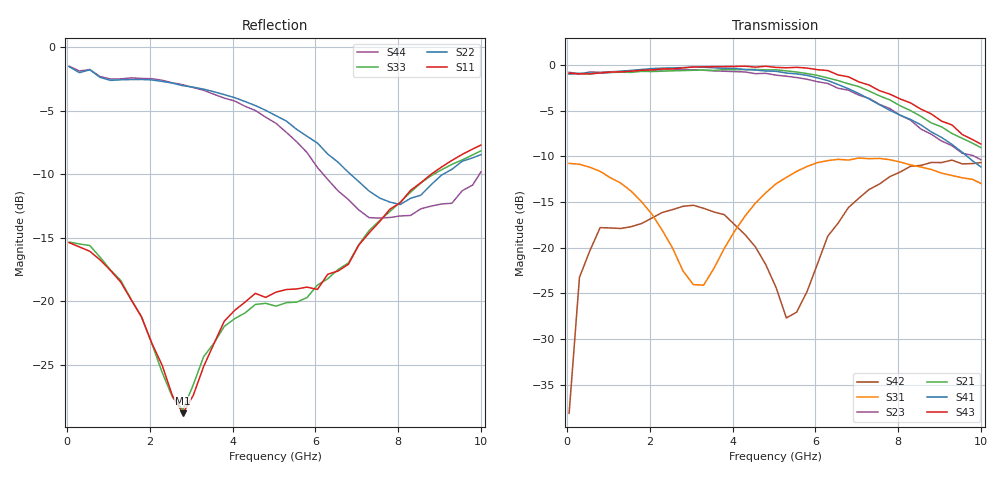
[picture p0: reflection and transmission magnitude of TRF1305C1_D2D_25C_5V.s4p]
! Created Tue Jun 24 22:55:10 2025
# hz S ma R 50
! 4 Port Network Data from SP1.SP block
! PORT[1] = INP
! PORT[2] = OUTM
! PORT[3] = INM
! PORT[4] = OUTP
! freq  magS11  angS11  magS12  angS12  magS13  angS13  magS14  angS14
!  magS21  angS21  magS22  angS22  magS23  angS23  magS24  angS24
!  magS31  angS31  magS32  angS32  magS33  angS33  magS34  angS34
!  magS41  angS41  magS42  angS42  magS43  angS43  magS44  angS44
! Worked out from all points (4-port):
!   41 points, 50 MHz to 10 GHz, reference 50 ohm
!   strongest paths, dB at 50 MHz, 2.55 GHz, 5.05 GHz, 7.55 GHz, 10 GHz:
!     S43: -0.9, -0.4, -0.3, -2.8, -8.7
!     S41: -1.0, -0.3, -0.7, -4.3, -11.2
!     S21: -0.9, -0.6, -0.5, -3.4, -9.0
!     S23: -0.8, -0.5, -1.1, -4.3, -10.4
!     S31: -10.8, -20.0, -13.0, -10.2, -13.0
!     S42: -38.1, -15.8, -24.4, -13.0, -10.7
!   lowest |S11| = -28.8 dB at 2.8 GHz (marker M1), VSWR 1.08, Z = 53.6 - j1.19 ohm
!   |S11| at or under -10 dB: start of sweep to 8.804 GHz
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5e7  0.1699 -1.5  0.004897 20.4  0.2954 -2.0  0.001261 -133.2
     0.8981 178.1  0.8368 178.4  0.9136 -2.0  0.01182 113.1
     0.2894 -2.0  0.00399 98.6  0.1708 -0.8  0.002537 18.8
     0.8926 -1.9  0.0124 122.8  0.9028 177.5  0.8406 178.9
5.5e8  0.1571 -19.1  0.02789 65.3  0.2843 -21.0  0.01899 71.4
       0.8943 157.8  0.8135 164.5  0.9165 -21.4  0.09531 68.9
       0.2758 -20.8  0.02184 69.4  0.1655 -17.2  0.02609 63.2
       0.9017 -20.8  0.09612 68.0  0.8947 158.0  0.8156 166.4
2.8e9  0.03619 -17.8  0.05857 -19.5  0.07844 -128.2  0.03886 -43.8
       0.9327 63.8  0.7042 121.2  0.9438 -112.6  0.1678 -1.2
       0.07477 -129.9  0.04105 -47.5  0.0374 -7.6  0.06172 -15.9
       0.9682 -109.4  0.1686 -4.4  0.9645 65.5  0.7104 128.2
4.3e9  0.09906 17.4  0.07177 -59.6  0.1466 91.2  0.04265 -103.5
       0.9454 -0.4  0.6104 91.4  0.917 -175.3  0.1241 -46.2
       0.1489 88.7  0.04447 -105.4  0.08983 22.8  0.07748 -55.3
       0.9445 -174.0  0.118 -52.5  0.9861 2.4  0.5844 97.9
6.05e9  0.1112 3.5  0.09128 -108.9  0.2992 33.5  0.03464 175.1
        0.8776 -80.8  0.4189 58.9  0.8106 103.1  0.06619 111.8
        0.2923 31.5  0.03239 177.4  0.1157 16.1  0.09526 -106.3
        0.8507 104.2  0.08138 115.8  0.943 -78.0  0.3357 67.4
7.8e9  0.23 5.0  0.09386 -162.2  0.3115 -10.3  0.01487 108.2
       0.6444 -159.4  0.2454 69.6  0.5781 21.8  0.2387 45.5
       0.3032 -10.4  0.01806 113.4  0.2252 8.8  0.1016 -159.1
       0.5653 22.8  0.2449 47.7  0.6933 -155.9  0.2133 78.4
1e10  0.4112 -44.9  0.08396 134.3  0.2292 -45.2  0.006797 16.3
      0.3532 119.3  0.3771 68.6  0.3031 -67.0  0.2925 -5.4
      0.2249 -43.8  0.008593 61.0  0.3902 -39.6  0.08687 138.3
      0.2769 -66.0  0.2926 -3.2  0.3694 120.4  0.3221 65.5
